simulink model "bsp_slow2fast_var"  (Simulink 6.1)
settings: Solver=ode45  StartTime=0.0  StopTime=20.0  RelTol=1e-3

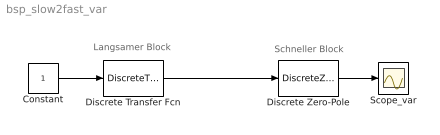
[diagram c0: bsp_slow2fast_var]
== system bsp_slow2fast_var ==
  note: Langsamer Block
  note: Schneller Block
  Constant : Constant
  Discrete Transfer Fcn : DiscreteTransferFcn  SampleTime=2
  Discrete Zero-Pole : DiscreteZeroPole  Poles=[0 0.5]  Gain=1
  Scope_var : Scope
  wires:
  Constant/1 -> Discrete Transfer Fcn/1
  Discrete Zero-Pole/1 -> Scope_var/1
  Discrete Transfer Fcn/1 -> Discrete Zero-Pole/1
